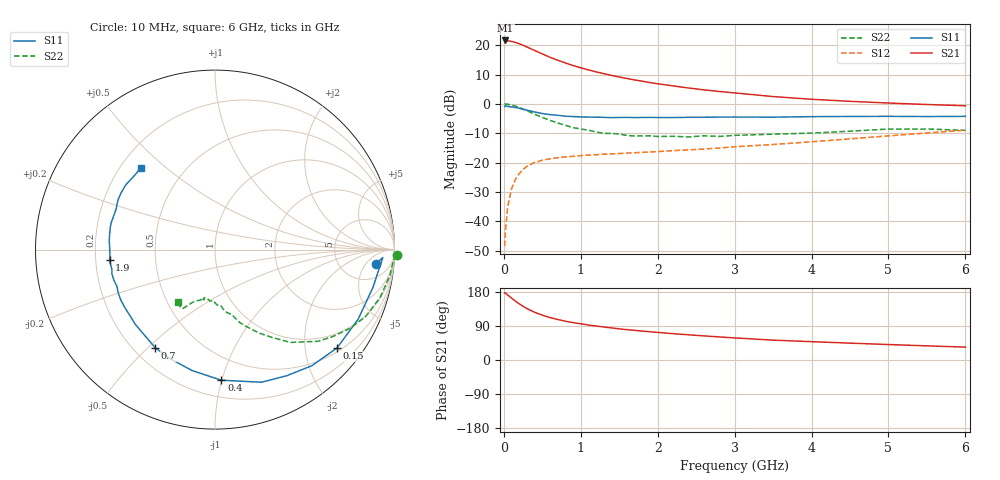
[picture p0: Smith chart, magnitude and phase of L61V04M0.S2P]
!  INFINEON TECHNOLOGIES Small Signal Semiconductors
! BFR380L3 , Si-NPN RF-Transistor in TSLP-3-1
!  Vce=1 V,  Ic=4 mA
! Common Emitter S-Parameters:  07. March 2005
#  GHz  S  MA  R  50
! f  S11  S21  S12  S22
! GHz  Mag  Ang  Mag  Ang  Mag  Ang  Mag  Ang
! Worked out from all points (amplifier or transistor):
!   36 points, 10 MHz to 6 GHz, reference 50 ohm
!   highest |S21| = 21.6 dB at 20 MHz (marker M1)
!   |S21| within 3 dB of that: start of sweep to 365.8 MHz
!   unconditionally stable (mu >= 1): 2.395 GHz to 4.872 GHz
!   at 250 MHz: K = 0.15, MSG = 21.1 dB, |S12| = -22.3 dB
!   at 1.4 GHz: K = 0.72, MSG = 13.3 dB, |S12| = -17.0 dB
!   at 6 GHz: K = 0.96, MSG = 4.2 dB, |S12| = -8.9 dB
!   S11 on the Smith chart (normalised r, x): 10 MHz: 11, -9; 150 MHz: 0.59, -2.72; 400 MHz: 0.32, -1.00; 700 MHz: 0.28, -0.53; 1.9 GHz: 0.26, -0.05; 6 GHz: 0.28, +0.41
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0.01  0.8978 -5.1  11.99 176.7  0.0038 87.4  1.012 -1.7
0.02  0.9362 -2.7  12 176.9  0.0068 87.1  0.9959 -3.4
0.05  0.9051 -13.4  11.88 171.5  0.0177 83.9  0.9854 -8.3
0.1  0.8869 -25.9  11.53 163.4  0.0359 76.8  0.9578 -16.2
0.15  0.8732 -38.9  11.14 155.4  0.0517 70.0  0.9192 -23.9
0.2  0.8423 -50.2  10.55 148.1  0.0652 64.8  0.8721 -30.1
0.25  0.8084 -60.4  9.935 141.8  0.077 59.3  0.8153 -36.5
0.3  0.783 -70.7  9.284 135.7  0.0866 55.1  0.7669 -41.8
0.4  0.7286 -87.2  8.116 125.9  0.1008 48.4  0.6672 -50.8
0.5  0.6859 -100.7  7.087 118.4  0.11 43.9  0.5875 -56.7
0.6  0.6571 -112.4  6.214 111.9  0.1165 40.7  0.5251 -62.2
0.7  0.6404 -121.3  5.533 106.9  0.1218 38.5  0.4738 -66.7
0.9  0.6088 -136.9  4.493 98.6  0.1284 35.8  0.3943 -73.9
1.1  0.5972 -147.2  3.785 92.3  0.1347 35.8  0.3575 -79.2
1.4  0.5836 -159.3  3.047 84.7  0.1409 36.2  0.3146 -85.2
1.9  0.5901 -174.2  2.304 74.5  0.1519 39.4  0.2871 -95.7
2.2  0.5865 179.3  2.023 69.5  0.1602 41.8  0.2812 -97.8
2.8  0.5963 168.2  1.628 60.9  0.1776 47.1  0.2797 -105.9
3.5  0.5952 157.8  1.333 52.4  0.2037 51.0  0.3055 -110.6
4.5  0.6114 149.0  1.106 44.5  0.2547 56.4  0.3431 -115.7
5.5  0.6094 138.5  0.977 37.3  0.3202 57.4  0.374 -121.2
6  0.614 132.4  0.929 34.0  0.3571 56.6  0.355 -125.0
